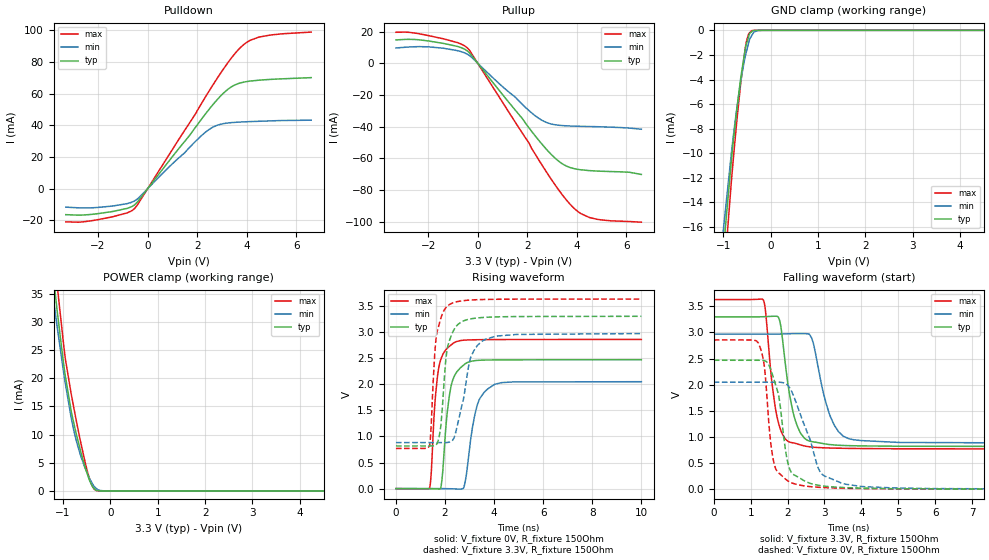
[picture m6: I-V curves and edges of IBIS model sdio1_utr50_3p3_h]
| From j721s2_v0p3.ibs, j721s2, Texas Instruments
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|   utr50_3p3_h
[Model]   sdio1_utr50_3p3_h
Model_type   I/O
Polarity   Non-Inverting
Enable   Active-High
Vinl = 0
Vinh = 0.8
Vmeas = 1.65
Vref = 3.3
Cref = 2pF
Rref = 100000
|   typ   min   max
C_comp   2.899pF   2.696pF   3.031pF
[Voltage Range]   3.3   2.97   3.63
[Temperature Range]   27   150   -40
[Pullup Reference]   3.3   2.97   3.63
[Pulldown Reference]   0   0   0
[Power Clamp Reference]   3.3   2.97   3.63
[GND Clamp Reference]   0   0   0
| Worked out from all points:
|   slope of the pulldown table from 0 to 0.495 V, typ, clamps not added: 49.2 ohm
|   slope of the pullup table from 0 to 0.495 V, typ, clamps not added: 50.3 ohm
|   GND clamp passes 1 mA (typ) near -0.50 V on its own axis
|   POWER clamp passes 1 mA (typ) near -0.39 V on its own axis
|   falling waveform, V_fixture 3.3V, R_fixture 150Ohm: 20-80 % time 337ps typ, 448ps min, 280ps max; typ from 3.3 V to 0.817 V
|   rising waveform, V_fixture 0V, R_fixture 150Ohm: 20-80 % time 319ps typ, 432ps min, 265ps max; typ from 0 V to 2.47 V
|   rising waveform, V_fixture 3.3V, R_fixture 150Ohm: 20-80 % time 310ps typ, 538ps min, 258ps max; typ from 0.817 V to 3.3 V
|   falling waveform, V_fixture 0V, R_fixture 150Ohm: 20-80 % time 325ps typ, 587ps min, 230ps max; typ from 2.47 V to 0 V
[Pulldown]
|   Voltage   I(typ)   I(min)   I(max)
-3.3V     -16.37mA   -11.62mA   -20.9mA
-2.092V   -15.89mA   -11.91mA   -19.74mA
-627mV    -11.19mA   -8.446mA   -13.78mA
-399.3mV  -8.123mA   -6.286mA   -9.93mA
2.006V    40.33mA    31.04mA    49.32mA
2.472V    49.92mA    37.27mA    61.41mA
2.779V    55.67mA    39.85mA    68.95mA
3.175V    61.91mA    41.34mA    78.12mA
3.749V    66.76mA    42.07mA    89.12mA
4.125V    67.88mA    42.33mA    93.49mA
4.481V    68.46mA    42.53mA    95.61mA
6.6V      70.08mA    43.23mA    98.81mA
[GND Clamp]
|   Voltage   I(typ)   I(min)   I(max)
-3.3V     -160mA     -119.4mA   -217mA
-1.033V   -19.39mA   -17.52mA   -22.42mA
-825mV    -10.43mA   -9.877mA   -12.11mA
-716.1mV  -6.541mA   -6.437mA   -7.501mA
-627mV    -3.775mA   -4.073mA   -4.143mA
-537.9mV  -1.565mA   -2.149mA   -1.561mA
-508.2mV  -1.103mA   -1.7mA     -875.2uA
-468.6mV  -579.1uA   -1.102mA   -332.1uA
-399.3mV  -111.6uA   -430.9uA   -25.71uA
-349.8mV  -18.88uA   -131.5uA   -5.144uA
-171.6mV  -88.29nA   -2.801uA   -107.4nA
6.6V      0A         0A         0A
[Pullup]
|   Voltage   I(typ)   I(min)   I(max)
-3.3V     14.73mA    9.638mA    19.55mA
-1.993V   14.07mA    10.37mA    17.48mA
-518.1mV  8.792mA    6.465mA    10.89mA
-280.5mV  5.597mA    4.208mA    6.944mA
2.006V    -39.52mA   -29.05mA   -48.98mA
2.501V    -49.39mA   -35.16mA   -62mA
3.194V    -60.92mA   -39mA      -78.43mA
3.472V    -64.04mA   -39.41mA   -84.28mA
3.887V    -66.53mA   -39.71mA   -91.59mA
4.155V    -67.25mA   -39.83mA   -94.87mA
4.778V    -68.04mA   -40.04mA   -98.4mA
6.6V      -70.21mA   -41.65mA   -100.3mA
[POWER Clamp]
|   Voltage   I(typ)   I(min)   I(max)
-3.3V     224.5mA    191.3mA    262.6mA
-1.211V   38.57mA    34.7mA     44.22mA
-1.132V   32.63mA    29.7mA     37.31mA
-1.122V   31.9mA     29.08mA    36.46mA
-953.7mV  20.54mA    19.22mA    23.62mA
-825mV    14.09mA    12.89mA    17.14mA
-765.6mV  11.78mA    10.49mA    14.49mA
-636.9mV  7.356mA    6.549mA    9.056mA
-478.5mV  2.813mA    2.955mA    3.268mA
-399.3mV  1.162mA    1.587mA    1.168mA
-290.4mV  108.5uA    386.4uA    43.38uA
6.6V      0A         0A         0A
[Ramp]
R_load = 150
|   typ   min   max
dV/dt_r   1.48067/3.18947e-10   1.22788/4.29223e-10   1.71387/2.64805e-10
dV/dt_f   1.48934/3.37023e-10   1.25229/4.4339e-10   1.71577/2.80464e-10
[Falling Waveform]
V_fixture = 3.3V
V_fixture_min = 2.97V
V_fixture_max = 3.63V
R_fixture = 150Ohm
C_fixture = 0F
|   Time   V(typ)   V(min)   V(max)
0s        3.3V       2.969V     3.63V
1.345ns   3.302V     2.969V     3.621V
1.6ns     3.311V     2.969V     1.909V
1.775ns   3.254V     2.97V      1.218V
2.055ns   1.816V     2.976V     902.3mV
2.33ns    1.103V     2.98V      851.6mV
2.655ns   910.8mV    2.894V     806.8mV
3.155ns   853.7mV    1.401V     788mV
3.66ns    833.8mV    966.1mV    781.1mV
10ns      817.4mV    882mV      770.1mV
[Rising Waveform]
V_fixture = 0V
V_fixture_min = 0V
V_fixture_max = 0V
R_fixture = 150Ohm
C_fixture = 0F
|   Time   V(typ)   V(min)   V(max)
0s        487.6uV    1.212mV    303.7uV
1.37ns    252.8uV    775.7uV    7.437mV
1.6ns     -2.622mV   584.1uV    1.705V
1.815ns   2.839mV    597.1uV    2.453V
2.115ns   1.553V     -812.6uV   2.699V
2.36ns    2.132V     -3.905mV   2.792V
2.765ns   2.369V     22.32mV    2.842V
3.385ns   2.457V     1.693V     2.852V
4.025ns   2.465V     1.998V     2.854V
10ns      2.468V     2.048V     2.857V
[Rising Waveform]
V_fixture = 3.3V
V_fixture_min = 2.97V
V_fixture_max = 3.63V
R_fixture = 150Ohm
C_fixture = 0F
|   Time   V(typ)   V(min)   V(max)
0s        817.4mV    882mV      770.1mV
1.36ns    817.2mV    881.8mV    812.1mV
1.65ns    845.7mV    881.7mV    2.927V
1.83ns    1.202V     881.7mV    3.262V
2.03ns    2.449V     882.1mV    3.461V
2.195ns   2.855V     892.2mV    3.529V
2.445ns   3.102V     1.093V     3.575V
3.045ns   3.25V      2.51V      3.611V
3.525ns   3.276V     2.828V     3.621V
10ns      3.3V       2.969V     3.63V
[Falling Waveform]
|Gnd
V_fixture = 0V
V_fixture_min = 0V
V_fixture_max = 0V
R_fixture = 150Ohm
C_fixture = 0F
|   Time   V(typ)   V(min)   V(max)
0s        2.468V     2.048V     2.857V
1.205ns   2.468V     2.048V     2.803V
1.37ns    2.461V     2.048V     2.357V
1.525ns   2.326V     2.048V     1.013V
1.635ns   2.093V     2.048V     491.6mV
1.98ns    598.2mV    2.008V     173.6mV
2.115ns   311.1mV    1.865V     121.2mV
2.87ns    70.09mV    349mV      34.99mV
3.485ns   32.7mV     111mV      17.89mV
10ns      486.9uV    1.212mV    303.7uV
